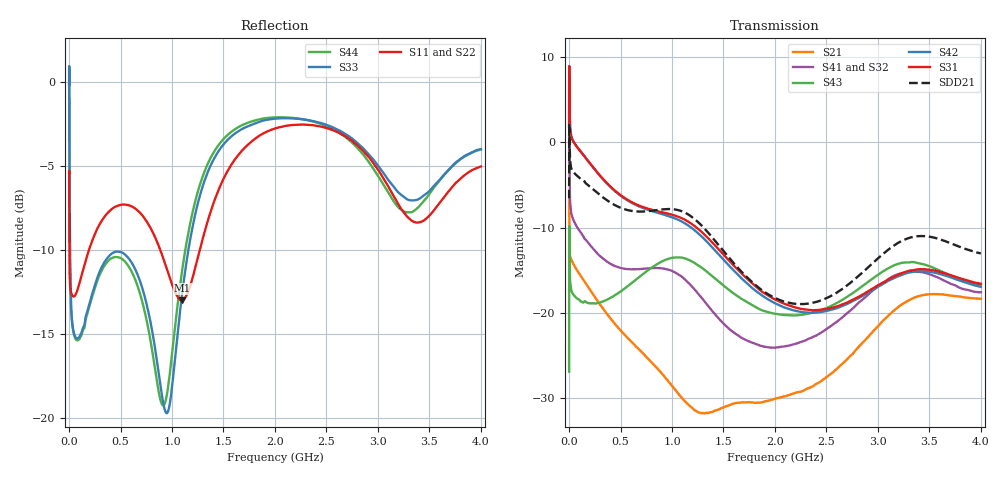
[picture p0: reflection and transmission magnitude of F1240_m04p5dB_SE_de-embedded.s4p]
! Integrated Device Technology
! Corporate Headquarters
! 6024 Silver Creek Valley Road
! San Jose, CA 95138  USA
! Phone:  1-408-284-8200
! Toll Free:  1-800-223-1366
! Webpage:  http://www.idt.com/
! Timing and RF Division
! 515 Groton Road, Suite 102
! Westford, MA 01886-6024
! Device:  F1240
! Description: Dual Intermediate Frequency Digital Variable Gain Amplifier
! Frequency:  10.0 -  500.00 MHz
! Package:  5x5 mm QFN Plastic Package: 32 pin
! Ports:  8 RF, 20 DC
!  Pin  1  = GA3 / Data  Pin 17  = RF OUT_B+
!  Pin  2  = GA4 / CLK  Pin 18  = RF OUT_B-
!  Pin  3  = GA5  Pin 19  = STBY_B
!  Pin  4  = VMODE  Pin 20  = Ground
!  Pin  5  = No Connect  Pin 21  = Ground
!  Pin  6  = GB5  Pin 22  = STB_A
!  Pin  7  = GB4  Pin 23  = RF OUT_A-  = Port 4
!  Pin  8  = GB3  Pin 24  = RF OUT_A+  = Port 3
!  Pin  9  = GB2  Pin 25  = GA0
!  Pin 10  = GB1  Pin 26  = ISET_A
!  Pin 11  = RF IN_B+  Pin 27  = VCC
!  Pin 12  = RF IN_B-  Pin 28  = Ground
!  Pin 13  = Ground  Pin 29  = RF IN_A-  = Port 2
!  Pin 14  = VCC  Pin 30  = RF IN_A+  = Port 1
!  Pin 15  = ISET_B  Pin 31  = GA1
!  Pin 16  = GB0  Pin 32  = GA2 / CSb
! Gain  = +19.5 dB
! State  = 1
! Voltage  = +5.00 V
! Current  = 85.292 mA (one channel only)
! Temperture  =  +25 C
! Test Date  =  2017-10-18
! Board  =  EB4031
! Data:  The device was measured on a custom evaluation board which has
!  individual transmission lines to the RF pins.  Data was collected
!  using a calibrated network analyzer.  The evaluation board was
!  de-embedded using Automatic Fixture Removal.
!  The reference plane is the edge of the package pin.
!  Only Channel A was measured.
!  This data is in single-ended operation.  If your needs are balanced
!  or differential S-parameters then this file needs to be used a
!  linear simulator.
! File Date:  2017-11-10  MJV
! Note:
!  Integrated Device Technology supplies this data as a sample of measured
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# Hz S dB R 100
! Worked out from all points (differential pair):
!   410 points, 500 kHz to 4 GHz, reference 100 ohm
!   strongest paths, dB at 500 kHz, 930 MHz, 1.96 GHz, 2.98 GHz, 4 GHz:
!     S31: 1.7, -8.3, -18.2, -16.9, -16.6
!     S42: 1.7, -8.5, -18.6, -17.1, -16.9
!     S43: -26.9, -13.8, -20.0, -15.7, -16.7
!     S41: -2.4, -14.8, -24.0, -17.1, -17.6
!     S32: -2.4, -15.0, -24.0, -17.4, -18.0
!     S21: -6.8, -27.5, -30.2, -21.8, -18.3
!   taken as a pair (ports 1,2 in; 3,4 out), SDD21 dB: -6.6, -7.8, -18.0, -13.8, -13.0
!   lowest |S11| = -13.0 dB at 1.1 GHz (marker M1), VSWR 1.58, Z = 64.8 - j11.3 ohm
!   |S11| at or under -10 dB: 3.075 MHz to 193.2 MHz (190.1 MHz wide, 194 % of centre); 885.7 MHz to 1.27 GHz (383.9 MHz wide, 35.6 % of centre)
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500000  -5.40 -5.6  -6.82 -5.9  -31.06 78.9  -35.14 77.4
        -6.83 -5.9  -5.39 -5.6  -35.11 76.2  -31.05 80.2
        1.74 -109.4  -2.42 -111.7  -0.18 0.3  -26.86 -40.3
        -2.45 -110.6  1.75 -108.3  -26.86 -40.5  -0.19 2.6
2000000  -7.80 -31.5  -9.67 -31.9  -22.32 24.2  -27.17 6.3
         -9.68 -31.9  -7.77 -31.6  -27.14 6.1  -22.31 24.5
         8.39 179.5  3.49 161.9  -0.17 -52.5  -9.79 -143.3
         3.45 162.2  8.40 179.8  -9.79 -143.3  -0.22 -52.2
4000000  -10.92 -26.7  -12.64 -21.8  -22.94 6.3  -30.25 -12.3
         -12.64 -21.9  -10.92 -27.0  -30.21 -12.5  -22.94 6.4
         5.02 157.9  -2.32 139.0  -4.68 -86.0  -12.53 173.5
         -2.36 139.2  5.02 158.1  -12.53 173.5  -4.73 -86.0
3.9e8  -7.70 -136.8  -20.44 -105.0  -27.07 -82.9  -36.28 -68.3
       -20.45 -105.0  -7.61 -137.9  -36.39 -66.7  -27.23 -83.2
       -5.05 56.9  -14.23 9.4  -10.36 -163.4  -18.38 42.7
       -14.16 8.6  -5.11 55.7  -18.31 42.3  -10.59 -164.0
1.1e9  -13.01 -158.2  -30.29 153.0  -26.24 139.4  -33.23 177.1
       -29.99 152.2  -12.98 -156.7  -33.22 -178.4  -27.18 139.3
       -8.92 -108.0  -16.01 160.0  -12.53 -106.6  -13.70 -147.3
       -15.79 154.9  -9.32 -110.4  -13.52 -147.3  -11.15 -107.5
2.85e9  -4.07 106.1  -23.54 -24.0  -27.38 -150.8  -29.65 -135.4
        -23.51 -24.1  -3.85 106.7  -30.33 -122.7  -28.70 -144.6
        -17.86 -65.3  -18.77 -148.3  -3.91 103.5  -17.65 -80.1
        -18.44 -159.4  -18.01 -62.2  -16.84 -78.0  -4.28 96.7
4e9  -5.04 -131.0  -18.35 113.3  -26.06 -36.5  -27.06 -20.9
     -18.34 113.2  -4.73 -129.7  -27.76 -6.2  -27.93 -28.5
     -16.57 42.7  -17.99 -56.7  -4.01 -133.6  -18.08 63.8
     -17.57 -70.8  -16.94 48.6  -16.69 56.3  -4.03 -143.3
